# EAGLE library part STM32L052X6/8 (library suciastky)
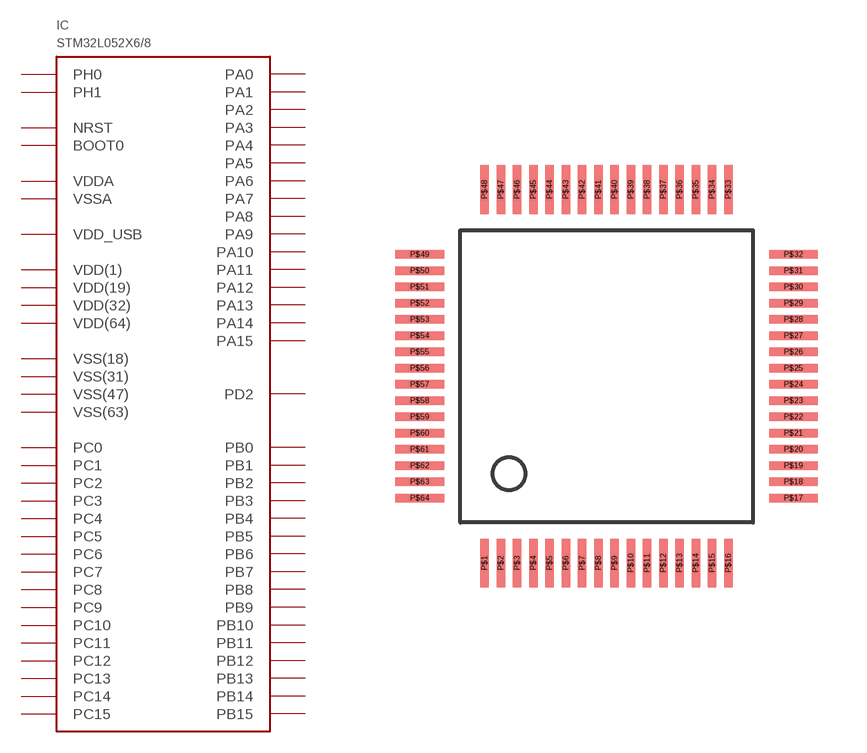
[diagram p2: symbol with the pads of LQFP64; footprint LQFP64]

Designator prefix IC

## STM32L052X6/8  [LQFP64]
P$1  VDD(1)  pwr
P$2  PC13
P$3  PC14
P$4  PC15
P$5  PH0  in
P$6  PH1  out
P$7  NRST
P$8  PC0
P$9  PC1
P$10  PC2
P$11  PC3
P$12  VSSA  pwr
P$13  VDDA  pwr
P$14  PA0
P$15  PA1
P$16  PA2
P$17  PA3
P$18  VSS(18)  pwr
P$19  VDD(19)  pwr
P$20  PA4
P$21  PA5
P$22  PA6
P$23  PA7
P$24  PC4
P$25  PC5
P$26  PB0
P$27  PB1
P$28  PB2
P$29  PB10
P$30  PB11
P$31  VSS(31)  pwr
P$32  VDD(32)  pwr
P$33  PB12
P$34  PB13
P$35  PB14
P$36  PB15
P$37  PC6
P$38  PC7
P$39  PC8
P$40  PC9
P$41  PA8
P$42  PA9
P$43  PA10
P$44  PA11
P$45  PA12
P$46  PA13
P$47  VSS(47)  pwr
P$48  VDD_USB  pwr
P$49  PA14
P$50  PA15
P$51  PC10
P$52  PC11
P$53  PC12
P$54  PD2
P$55  PB3
P$56  PB4
P$57  PB5
P$58  PB6
P$59  PB7
P$60  BOOT0
P$61  PB8
P$62  PB9
P$63  VSS(63)  pwr
P$64  VDD(64)  pwr

## Footprint LQFP64 (pad centres in mm)
smd 0.254 x 1.5: P$1 -3.75,-5.75; P$2 -3.25,-5.75; P$3 -2.75,-5.75; P$4 -2.25,-5.75; P$5 -1.75,-5.75; P$6 -1.25,-5.75; P$7 -0.75,-5.75; P$8 -0.25,-5.75; P$9 0.25,-5.75; P$10 0.75,-5.75; P$11 1.25,-5.75; P$12 1.75,-5.75; P$13 2.25,-5.75; P$14 2.75,-5.75; P$15 3.25,-5.75; P$16 3.75,-5.75; P$33 3.75,5.75; P$34 3.25,5.75; P$35 2.75,5.75; P$36 2.25,5.75; P$37 1.75,5.75; P$38 1.25,5.75; P$39 0.75,5.75; P$40 0.25,5.75; P$41 -0.25,5.75; P$42 -0.75,5.75; P$43 -1.25,5.75; P$44 -1.75,5.75; P$45 -2.25,5.75; P$46 -2.75,5.75; P$47 -3.25,5.75; P$48 -3.75,5.75
smd 1.5 x 0.254: P$17 5.75,-3.75; P$18 5.75,-3.25; P$19 5.75,-2.75; P$20 5.75,-2.25; P$21 5.75,-1.75; P$22 5.75,-1.25; P$23 5.75,-0.75; P$24 5.75,-0.25; P$25 5.75,0.25; P$26 5.75,0.75; P$27 5.75,1.25; P$28 5.75,1.75; P$29 5.75,2.25; P$30 5.75,2.75; P$31 5.75,3.25; P$32 5.75,3.75; P$49 -5.75,3.75; P$50 -5.75,3.25; P$51 -5.75,2.75; P$52 -5.75,2.25; P$53 -5.75,1.75; P$54 -5.75,1.25; P$55 -5.75,0.75; P$56 -5.75,0.25; P$57 -5.75,-0.25; P$58 -5.75,-0.75; P$59 -5.75,-1.25; P$60 -5.75,-1.75; P$61 -5.75,-2.25; P$62 -5.75,-2.75; P$63 -5.75,-3.25; P$64 -5.75,-3.75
